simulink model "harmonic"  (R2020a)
settings: Solver=ode45  StartTime=0.0  StopTime=10.0  RelTol=1e-3  EnableMultiTasking=on

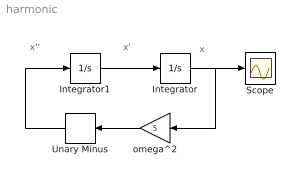
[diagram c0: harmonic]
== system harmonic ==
  note: x'
  note: x''
  note: x
  note: .
  Integrator : Integrator  InitialCondition=3
  Integrator1 : Integrator
  Scope : Scope
  Unary Minus : UnaryMinus
  omega^2 : Gain  Gain=5  SaturateOnIntegerOverflow=on
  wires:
  Integrator1/1 -> Integrator/1
  Integrator/1 -> omega^2/1, Scope/1
  omega^2/1 -> Unary Minus/1
  Unary Minus/1 -> Integrator1/1
